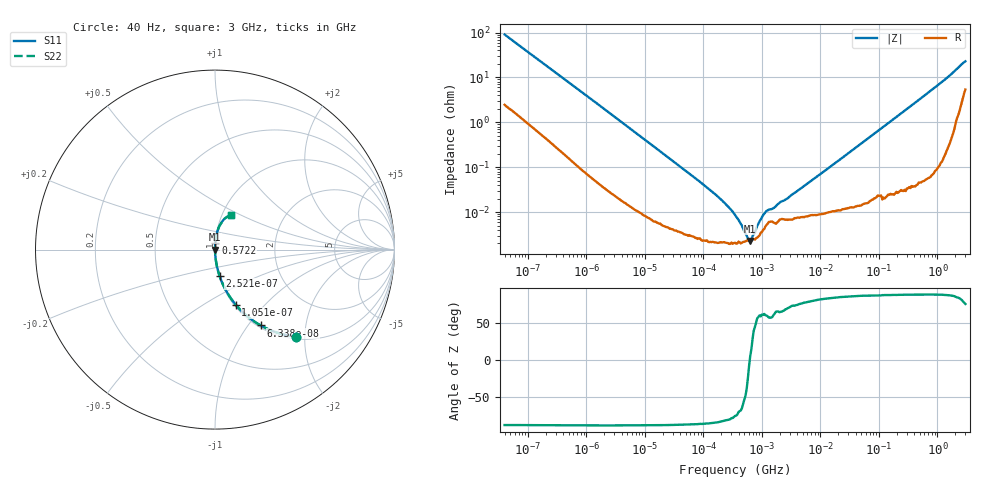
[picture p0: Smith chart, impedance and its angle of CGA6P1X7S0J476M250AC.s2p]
! S-parameter Generated by TDK Corporation
! Copyright(C) 2015 TDK Corporation.
! All Rights Reserved.
! TDK P/N: CGA6P1X7S0J476M250AC (Multilayer Ceramic Chip Capacitors)
! Property: C=47uF
! Size(LxWxT): 3.2x2.5x2.5mm, 0.126x0.098x0.098inches
! Model Type: s2p (Touchstone File Format Version 1.0)
! Frequency: DC=Yes Start=0.00004MHz Stop=3000MHz 396points Log-sweep
! Note: This model was converted from impedance.
! Model Generated on Jun. 23, 2015
! Hash(MD5):
! Port Assignments:
!  1 ---| |--- 2
! Applicable Conditions:
!  Temperature = 25 degC
!  DC Bias Voltage = 0 V
!  Small Signal Operation
! Terms and conditions regarding TDK Simulation Models
! (1)This simulation model is being provided solely for informational purposes. Please refer to the specifications of the products in terms of detailed characteristics of such products.
! (2)In no event shall TDK Corporation of any of its subsidiaries be liable for any loss or damage arising, directly or indirectly,
!  From any information contained in this simulation model, including, but not limited to loss or damages arising from any inaccuracies, omissions or errors in connection with such information.
! (3)Any and all copyrights on this simulation model are owned by TDK Corporation.
!  Duplication or redistribution of this simulation model without prior written permission from TDK Corporation is prohibited.
! (4)This simulation model is subject to any modification or change without any prior notice.
! (5)Neither TDK Corporation nor any of its subsidiaries shall make any warranty, express or implied,
!  Including but not limited to the correctness, implied warranties of merchantability and fitness for a particular purpose with respect to this simulation models.
! (6)The use of this simulation model shall be deemed to have consented to the terms and conditions hereof.
# MHz S MA R 50
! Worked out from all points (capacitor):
!   395 points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, 40 Hz to 3 GHz, reference 50 ohm
!   read as one part in series: C = 43.9 uF near 41.88 Hz
!   lowest |Z| = 2.29 mohm at 630.1 kHz (marker M1)
!   series resonance near 619.3 kHz, so ESL is about 1.5 nH
!   S11 on the Smith chart (normalised r, x): 40 Hz: 1.05, -1.81; 63.38 Hz: 1.03, -1.15; 105.1 Hz: 1.02, -0.70; 252.1 Hz: 1.01, -0.30; 572.2 MHz: 1.00, +0.08; 3 GHz: 1.11, +0.45
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4e-05  0.6626 -47.0  0.7313 41.5  0.7313 41.5  0.6626 -47.0
6.337743e-05  0.4931 -58.9  0.857 29.5  0.857 29.5  0.4931 -58.9
0.000105147  0.3288 -69.4  0.9361 19.2  0.9361 19.2  0.3288 -69.4
0.0001519485  0.2371 -74.9  0.9658 13.7  0.9658 13.7  0.2371 -74.9
0.0002520917  0.1482 -80.2  0.9856 8.5  0.9856 8.5  0.1482 -80.2
0.000834128  0.04703 -86.3  0.998 2.7  0.998 2.7  0.04703 -86.3
0.01739424  0.002364 -88.5  0.9999 0.1  0.9999 0.1  0.002364 -88.5
0.1046927  0.0003912 -86.6  1 0.0  1 0.0  0.0003912 -86.6
0.1818721  0.0002144 -84.5  1 0.0  1 0.0  0.0002144 -84.5
0.3159481  0.0001025 -79.0  1 0.0  1 0.0  0.0001025 -79.0
0.3464102  8.672e-05 -76.1  1 0.0  1 0.0  8.672e-05 -76.1
0.6301264  2.292e-05 5.3  1 -0.0  1 -0.0  2.292e-05 5.3
1.146211  9.935e-05 61.1  1 -0.0  1 -0.0  9.935e-05 61.1
1.315913  0.0001141 57.8  0.9999 -0.0  0.9999 -0.0  0.0001141 57.8
1.510739  0.000119 58.9  0.9999 -0.0  0.9999 -0.0  0.000119 58.9
2.084979  0.0001688 65.8  0.9999 -0.0  0.9999 -0.0  0.0001688 65.8
2.748062  0.000203 70.7  0.9999 -0.0  0.9999 -0.0  0.000203 70.7
7.22376  0.0005175 80.4  0.9999 -0.0  0.9999 -0.0  0.0005175 80.4
150.6385  0.01002 88.0  0.9997 -0.6  0.9997 -0.6  0.01002 88.0
572.2325  0.03768 87.1  0.9988 -2.2  0.9988 -2.2  0.03768 87.1
1808.253  0.1239 80.5  0.9873 -7.1  0.9873 -7.1  0.1239 80.5
3000  0.2127 64.5  0.9286 -11.9  0.9286 -11.9  0.2127 64.5
